FUNCTION_BLOCK FB_DO_IED_LD1_XCBR1_BlkCls EXTENDS FB_AcsiCommonControllableDataClass
VAR_INPUT
	ctlModel: FB_AcsiDATypeCtlModels := (fc:=ACSI_FC_CF, TrgOp:=ACSI_TrgOp_dchg, eValue:=E_AcsiCtlModels.StatusOnly, bLinkResult:=THIS^.AddDataToContainer(ipData:=ctlModel));
END_VAR
VAR
END_VAR

END_FUNCTION_BLOCK
